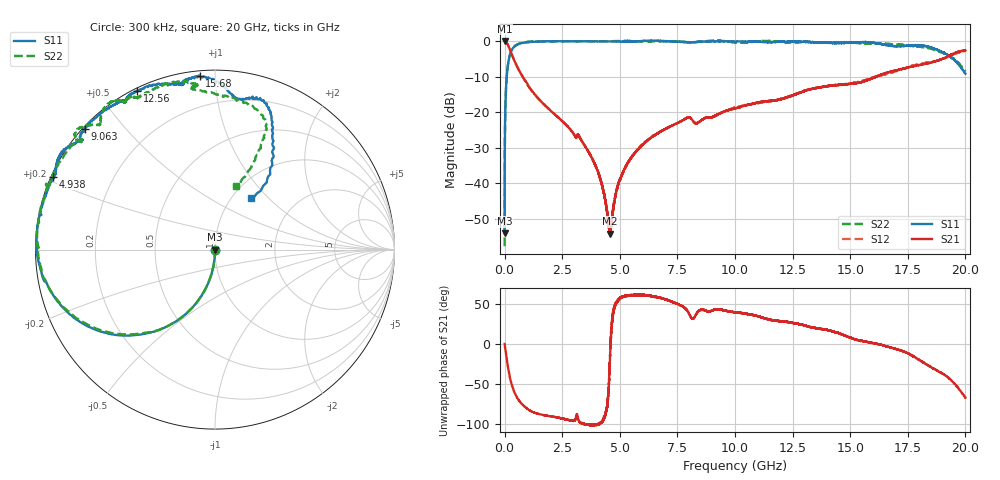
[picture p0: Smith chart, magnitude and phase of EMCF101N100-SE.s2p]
!EMCF101N100
!Johanson Technology Inc.
!www.johansontechnology.com
!Test Board Conditions:
!Substrate Type  RO4350B
!Substrate Thickness  6.6 mil
!Substrate Dk  3.66
!TL Type: GCPW
!TL Trace Width  13 mil
!TL Gap  7.5 mil
!PART MODE SINGLE ENDED (AKA BYPASS)
!DUT TOPOLOGY	SERIES-SHUNT
# MHz S  dB  R 50
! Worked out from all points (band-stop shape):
!   20001 points, 300 kHz to 20 GHz, reference 50 ohm
!   highest |S21| = 0.00 dB at 300 kHz (marker M1); lowest = -54.1 dB at 4.578 GHz (marker M2)
!   |S21| within 3 dB of the highest: start of sweep to 263.4 MHz; 19.7 GHz to end of sweep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
!   lowest |S11| = -54.1 dB at 300 kHz (marker M3), VSWR 1.00, Z = 50.2 - j0.123 ohm
!   |S11| at or under -10 dB: start of sweep to 92.97 MHz
!   |S22| runs from -57.7 to 0.2 dB; largest |S21 - S12| = 0.023
!   S11 on the Smith chart (normalised r, x): 300 kHz: 1.00, -0.00; 4.938 GHz: 0.00, +0.21; 9.063 GHz: 0.01, +0.39; 12.56 GHz: 0.01, +0.62; 15.68 GHz: 0.03, +0.92; 20 GHz: 1.22, +0.79
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0.3  -54.06 -38.2  0.00 -0.2  0.02 -0.2  -57.67 8.1
116.298  -8.29 -113.8  -0.72 -23.5  -0.71 -23.5  -8.33 -113.7
199.297  -4.72 -127.6  -1.86 -37.0  -1.84 -37.0  -4.76 -127.4
337.295  -2.18 -143.8  -4.18 -53.3  -4.16 -53.4  -2.21 -144.4
601.291  -0.81 -159.7  -7.91 -69.4  -7.91 -69.6  -0.79 -160.7
1015.285  -0.28 -169.7  -12.49 -81.3  -12.53 -81.4  -0.23 -174.2
3334.25  -0.04 167.3  -27.93 -98.3  -27.94 -98.6  -0.00 169.1
4092.239  -0.09 161.6  -37.49 -99.7  -37.44 -99.3  -0.04 162.0
4578.231  -0.07 157.9  -54.11 -15.9  -53.68 -14.3  -0.04 159.6
4938.226  -0.07 155.8  -40.11 54.6  -40.07 54.2  0.03 158.6
5612.216  -0.07 153.7  -31.78 60.4  -31.75 60.9  -0.01 159.1
6667.2  0.09 147.4  -25.87 57.8  -25.80 57.6  -0.04 154.3
7943.181  -0.31 140.6  -21.52 40.7  -21.48 40.9  -0.33 140.4
9063.164  -0.09 137.0  -21.24 41.9  -21.31 42.0  0.12 140.0
10000.15  -0.09 130.6  -18.91 39.2  -18.71 39.4  -0.37 133.6
12556.11  -0.13 116.1  -15.14 25.7  -15.00 25.7  -0.31 121.2
13334.1  -0.29 108.1  -13.44 20.3  -13.40 19.8  -0.33 118.1
15680.07  -0.28 95.0  -11.15 2.6  -10.91 2.2  -0.65 96.6
16667.05  -1.27 83.8  -8.74 -3.8  -9.10 -3.9  -0.83 98.1
18598.02  -1.99 66.7  -5.88 -30.4  -5.80 -31.8  -2.36 68.6
19431.01  -4.84 56.1  -3.67 -46.6  -3.87 -47.4  -4.67 65.6
20000  -9.16 55.1  -2.63 -66.8  -2.70 -66.1  -8.60 72.0
